(* Logix 5000 AddOnInstructionDefinition export CIP_Axis_Disable; software revision 34.01; part 3 of 4 *)
(* tags used below, declared in another part *)
   StateMachineErrorCode : INT;
   StateMachineErrorDescription : STRING;
   UpdatePeriod : DINT;
   Unwind : DINT;
   AxisControlWord : INT;
   AxisReadyToSwitchOn : BOOL;
   AxisSwitchedOn : BOOL;
   AxisOperationEnabled : BOOL;
   AxisFaulted : BOOL;
   AxisVoltageEnabled : BOOL;
   AxisQuickStop : BOOL;
   AxisSwitchOnDisabled : BOOL;
   AxisWarning : BOOL;
   AxisSTO : BOOL;
   AxisRemote : BOOL;
   AxisTargetReached : BOOL;
   AxisInternalLimitActive : BOOL;
   AxisHomeAttained : BOOL;
   AxisHomingError : BOOL;
   AxisMotionModeHoming : BOOL;
   AxisMotionModeCyclicPosition : BOOL;
   AxisFollowingError : BOOL;
   AxisStreamingActive : BOOL;
   ErrorEnumeratedValues : STRING[13];
   UpdatePeriodMsgSent : BOOL;
   UnwindMsgSent : BOOL;
   IsRotary : SINT;
(* CIP_Axis_State_Machine, continued *)

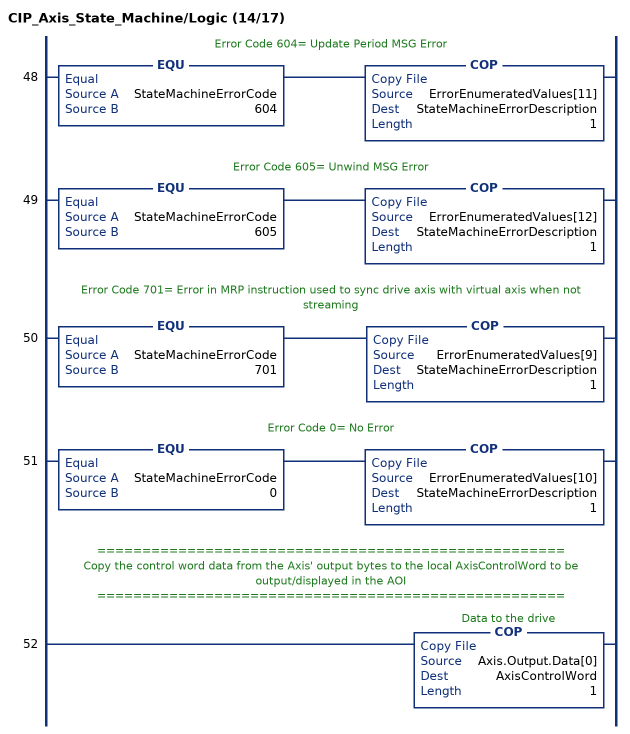
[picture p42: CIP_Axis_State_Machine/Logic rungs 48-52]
   // Error Code 604= Update Period MSG Error
   48: EQU(StateMachineErrorCode,604)COP(ErrorEnumeratedValues[11],StateMachineErrorDescription,1);
   // Error Code 605= Unwind MSG Error
   49: EQU(StateMachineErrorCode,605)COP(ErrorEnumeratedValues[12],StateMachineErrorDescription,1);
   // Error Code 701= Error in MRP instruction used to sync drive axis with virtual axis when not streaming
   50: EQU(StateMachineErrorCode,701)COP(ErrorEnumeratedValues[9],StateMachineErrorDescription,1);
   // Error Code 0= No Error
   51: EQU(StateMachineErrorCode,0)COP(ErrorEnumeratedValues[10],StateMachineErrorDescription,1);
   // ====================================================
   // Copy the control word data from the Axis' output bytes to the local AxisControlWord to be output/displayed in the AOI
   // ====================================================
   52: COP(Axis.Output.Data[0],AxisControlWord,1);
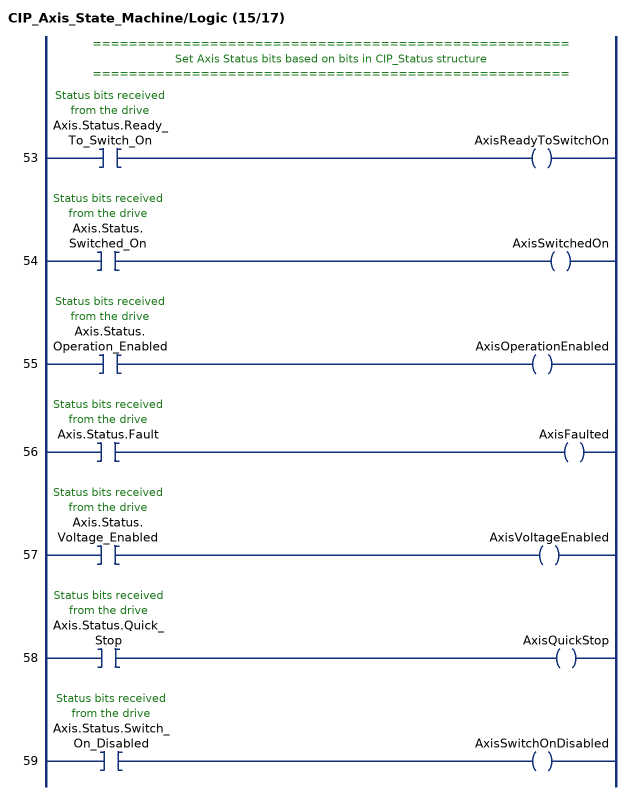
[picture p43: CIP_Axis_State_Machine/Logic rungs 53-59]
   // =====================================================
   // Set Axis Status bits based on bits in CIP_Status structure
   // =====================================================
   53: XIC(Axis.Status.Ready_To_Switch_On)OTE(AxisReadyToSwitchOn);
   54: XIC(Axis.Status.Switched_On)OTE(AxisSwitchedOn);
   55: XIC(Axis.Status.Operation_Enabled)OTE(AxisOperationEnabled);
   56: XIC(Axis.Status.Fault)OTE(AxisFaulted);
   57: XIC(Axis.Status.Voltage_Enabled)OTE(AxisVoltageEnabled);
   58: XIC(Axis.Status.Quick_Stop)OTE(AxisQuickStop);
   59: XIC(Axis.Status.Switch_On_Disabled)OTE(AxisSwitchOnDisabled);
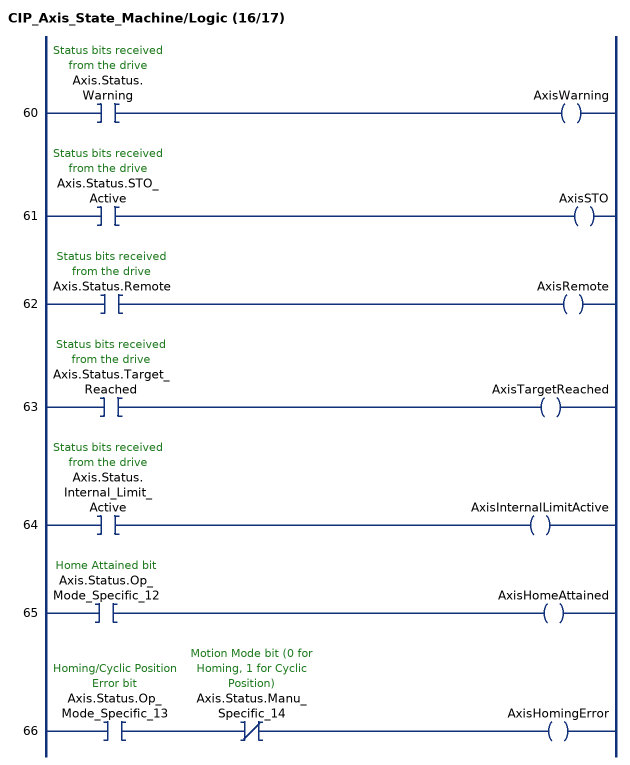
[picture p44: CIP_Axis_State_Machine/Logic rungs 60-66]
   60: XIC(Axis.Status.Warning)OTE(AxisWarning);
   61: XIC(Axis.Status.STO_Active)OTE(AxisSTO);
   62: XIC(Axis.Status.Remote)OTE(AxisRemote);
   63: XIC(Axis.Status.Target_Reached)OTE(AxisTargetReached);
   64: XIC(Axis.Status.Internal_Limit_Active)OTE(AxisInternalLimitActive);
   65: XIC(Axis.Status.Op_Mode_Specific_12)OTE(AxisHomeAttained);
   66: XIC(Axis.Status.Op_Mode_Specific_13)XIO(Axis.Status.Manu_Specific_14)OTE(AxisHomingError);
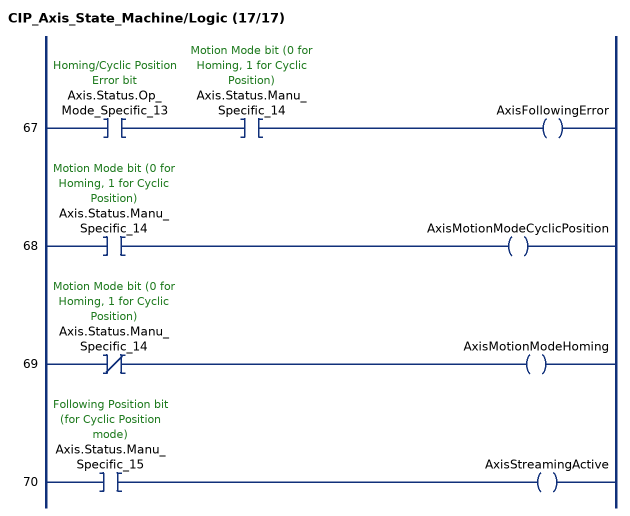
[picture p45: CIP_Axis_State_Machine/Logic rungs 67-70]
   67: XIC(Axis.Status.Op_Mode_Specific_13)XIC(Axis.Status.Manu_Specific_14)OTE(AxisFollowingError);
   68: XIC(Axis.Status.Manu_Specific_14)OTE(AxisMotionModeCyclicPosition);
   69: XIO(Axis.Status.Manu_Specific_14)OTE(AxisMotionModeHoming);
   70: XIC(Axis.Status.Manu_Specific_15)OTE(AxisStreamingActive);
END_ROUTINE

ROUTINE Prescan   (* ladder *)
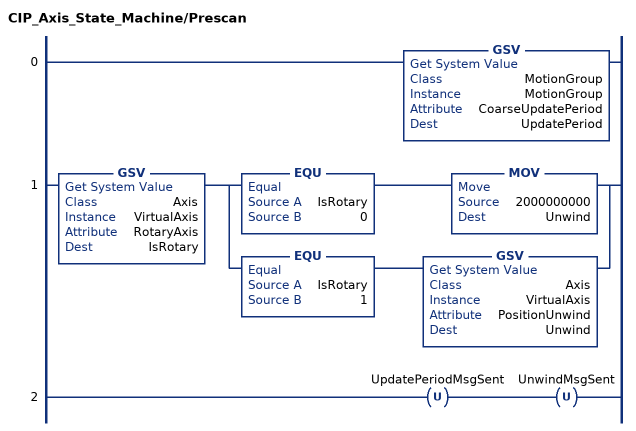
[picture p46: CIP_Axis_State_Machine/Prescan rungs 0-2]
   0: GSV(MotionGroup,MotionGroup,CoarseUpdatePeriod,UpdatePeriod);
   1: GSV(Axis,VirtualAxis,RotaryAxis,IsRotary)[EQU(IsRotary,0) MOV(2000000000,Unwind) ,EQU(IsRotary,1) GSV(Axis,VirtualAxis,PositionUnwind,Unwind) ];
   2: OTU(UpdatePeriodMsgSent)OTU(UnwindMsgSent);
END_ROUTINE
END_ADD_ON_INSTRUCTION

ADD_ON_INSTRUCTION CIP_Drive_Comms_Dual_Axis   (* revision 2.1, ExecutePrescan *)
// CIP Sync Drive Communications For AKD2G Dual Axis Drive
// Revision note:
// Changed local tag CycleStartTime from LINT to DINT[2]. Changed GSV destination and both COP instruction Source entries to use CycleStartTime[0] as a result of the change in data typing.
VAR_IN_OUT
   InputFromDrive : SINT[64]; {required}
   OutputToDrive : SINT[64]; {required}
   Axis1 : CIP_Axis; {required}
   Axis2 : CIP_Axis; {required}
   VirtualAxis1 : AXIS_VIRTUAL; {required}
   VirtualAxis2 : AXIS_VIRTUAL; {required}
   MotionGroup : MOTION_GROUP; {required}
   DynamicMap : CIP_DynamicMap; {required}
END_VAR
VAR
   CycleStartTime : DINT[2]; {access None}
   AxisPosition : DINT; {access None}
END_VAR

ROUTINE Logic   (* ladder *)
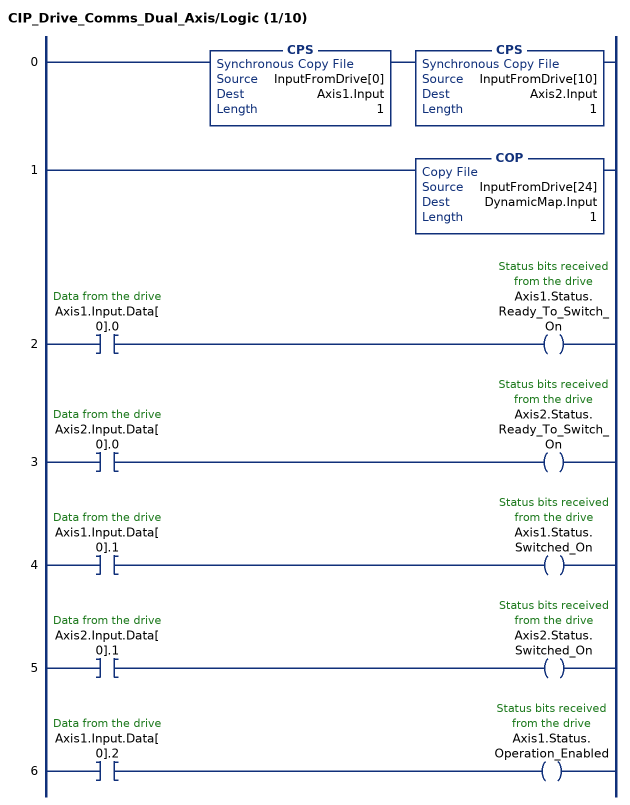
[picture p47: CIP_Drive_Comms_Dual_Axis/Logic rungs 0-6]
   0: CPS(InputFromDrive[0],Axis1.Input,1)CPS(InputFromDrive[10],Axis2.Input,1);
   1: COP(InputFromDrive[24],DynamicMap.Input,1);
   2: XIC(Axis1.Input.Data[0].0)OTE(Axis1.Status.Ready_To_Switch_On);
   3: XIC(Axis2.Input.Data[0].0)OTE(Axis2.Status.Ready_To_Switch_On);
   4: XIC(Axis1.Input.Data[0].1)OTE(Axis1.Status.Switched_On);
   5: XIC(Axis2.Input.Data[0].1)OTE(Axis2.Status.Switched_On);
   6: XIC(Axis1.Input.Data[0].2)OTE(Axis1.Status.Operation_Enabled);
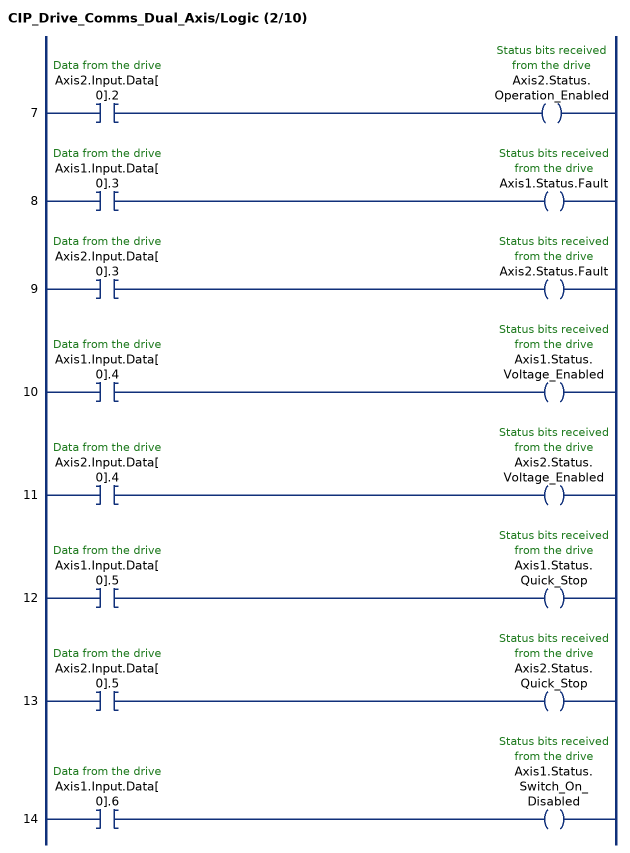
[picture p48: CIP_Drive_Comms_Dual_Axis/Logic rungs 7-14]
   7: XIC(Axis2.Input.Data[0].2)OTE(Axis2.Status.Operation_Enabled);
   8: XIC(Axis1.Input.Data[0].3)OTE(Axis1.Status.Fault);
   9: XIC(Axis2.Input.Data[0].3)OTE(Axis2.Status.Fault);
   10: XIC(Axis1.Input.Data[0].4)OTE(Axis1.Status.Voltage_Enabled);
   11: XIC(Axis2.Input.Data[0].4)OTE(Axis2.Status.Voltage_Enabled);
   12: XIC(Axis1.Input.Data[0].5)OTE(Axis1.Status.Quick_Stop);
   13: XIC(Axis2.Input.Data[0].5)OTE(Axis2.Status.Quick_Stop);
   14: XIC(Axis1.Input.Data[0].6)OTE(Axis1.Status.Switch_On_Disabled);
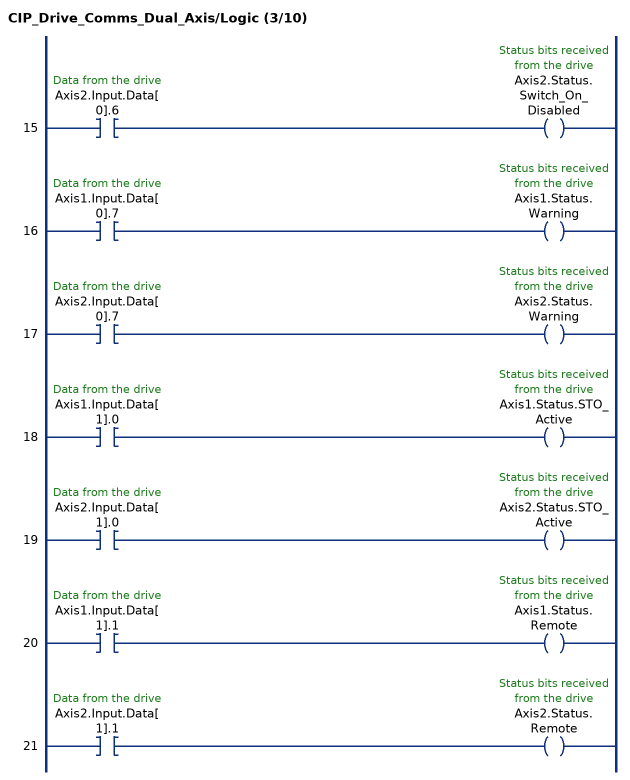
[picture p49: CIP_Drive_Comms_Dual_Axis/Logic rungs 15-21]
   15: XIC(Axis2.Input.Data[0].6)OTE(Axis2.Status.Switch_On_Disabled);
   16: XIC(Axis1.Input.Data[0].7)OTE(Axis1.Status.Warning);
   17: XIC(Axis2.Input.Data[0].7)OTE(Axis2.Status.Warning);
   18: XIC(Axis1.Input.Data[1].0)OTE(Axis1.Status.STO_Active);
   19: XIC(Axis2.Input.Data[1].0)OTE(Axis2.Status.STO_Active);
   20: XIC(Axis1.Input.Data[1].1)OTE(Axis1.Status.Remote);
   21: XIC(Axis2.Input.Data[1].1)OTE(Axis2.Status.Remote);
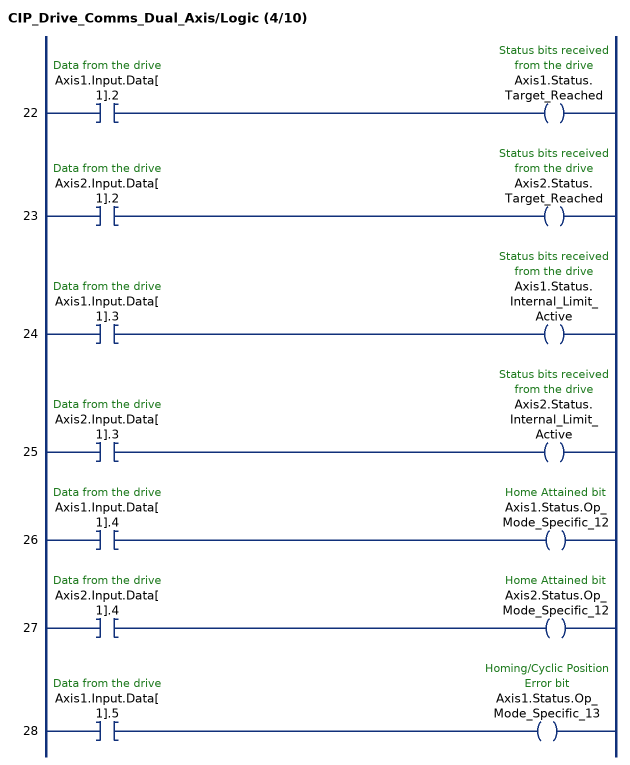
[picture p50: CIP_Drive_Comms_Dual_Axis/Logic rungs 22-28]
   22: XIC(Axis1.Input.Data[1].2)OTE(Axis1.Status.Target_Reached);
   23: XIC(Axis2.Input.Data[1].2)OTE(Axis2.Status.Target_Reached);
   24: XIC(Axis1.Input.Data[1].3)OTE(Axis1.Status.Internal_Limit_Active);
   25: XIC(Axis2.Input.Data[1].3)OTE(Axis2.Status.Internal_Limit_Active);
   26: XIC(Axis1.Input.Data[1].4)OTE(Axis1.Status.Op_Mode_Specific_12);
   27: XIC(Axis2.Input.Data[1].4)OTE(Axis2.Status.Op_Mode_Specific_12);
   28: XIC(Axis1.Input.Data[1].5)OTE(Axis1.Status.Op_Mode_Specific_13);
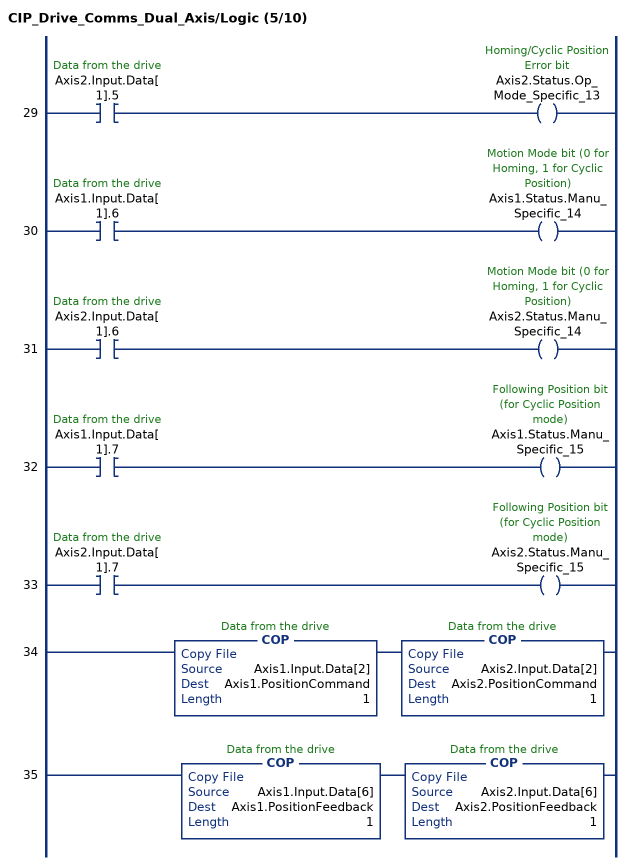
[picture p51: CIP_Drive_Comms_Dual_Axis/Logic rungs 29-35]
   29: XIC(Axis2.Input.Data[1].5)OTE(Axis2.Status.Op_Mode_Specific_13);
   30: XIC(Axis1.Input.Data[1].6)OTE(Axis1.Status.Manu_Specific_14);
   31: XIC(Axis2.Input.Data[1].6)OTE(Axis2.Status.Manu_Specific_14);
   32: XIC(Axis1.Input.Data[1].7)OTE(Axis1.Status.Manu_Specific_15);
   33: XIC(Axis2.Input.Data[1].7)OTE(Axis2.Status.Manu_Specific_15);
   34: COP(Axis1.Input.Data[2],Axis1.PositionCommand,1)COP(Axis2.Input.Data[2],Axis2.PositionCommand,1);
   35: COP(Axis1.Input.Data[6],Axis1.PositionFeedback,1)COP(Axis2.Input.Data[6],Axis2.PositionFeedback,1);
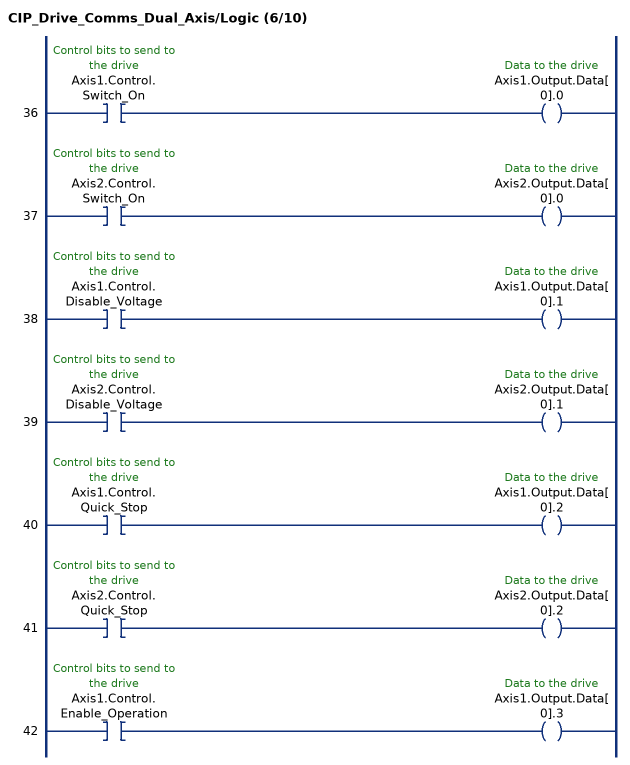
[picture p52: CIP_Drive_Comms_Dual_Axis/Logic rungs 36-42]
   36: XIC(Axis1.Control.Switch_On)OTE(Axis1.Output.Data[0].0);
   37: XIC(Axis2.Control.Switch_On)OTE(Axis2.Output.Data[0].0);
   38: XIC(Axis1.Control.Disable_Voltage)OTE(Axis1.Output.Data[0].1);
   39: XIC(Axis2.Control.Disable_Voltage)OTE(Axis2.Output.Data[0].1);
   40: XIC(Axis1.Control.Quick_Stop)OTE(Axis1.Output.Data[0].2);
   41: XIC(Axis2.Control.Quick_Stop)OTE(Axis2.Output.Data[0].2);
   42: XIC(Axis1.Control.Enable_Operation)OTE(Axis1.Output.Data[0].3);
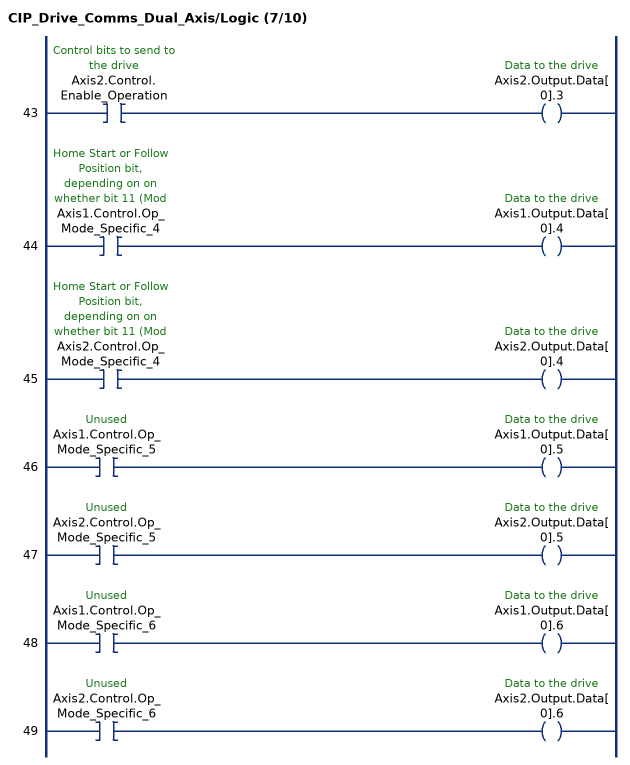
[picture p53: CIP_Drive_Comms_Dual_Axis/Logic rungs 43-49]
   43: XIC(Axis2.Control.Enable_Operation)OTE(Axis2.Output.Data[0].3);
   44: XIC(Axis1.Control.Op_Mode_Specific_4)OTE(Axis1.Output.Data[0].4);
   45: XIC(Axis2.Control.Op_Mode_Specific_4)OTE(Axis2.Output.Data[0].4);
   46: XIC(Axis1.Control.Op_Mode_Specific_5)OTE(Axis1.Output.Data[0].5);
   47: XIC(Axis2.Control.Op_Mode_Specific_5)OTE(Axis2.Output.Data[0].5);
   48: XIC(Axis1.Control.Op_Mode_Specific_6)OTE(Axis1.Output.Data[0].6);
   49: XIC(Axis2.Control.Op_Mode_Specific_6)OTE(Axis2.Output.Data[0].6);
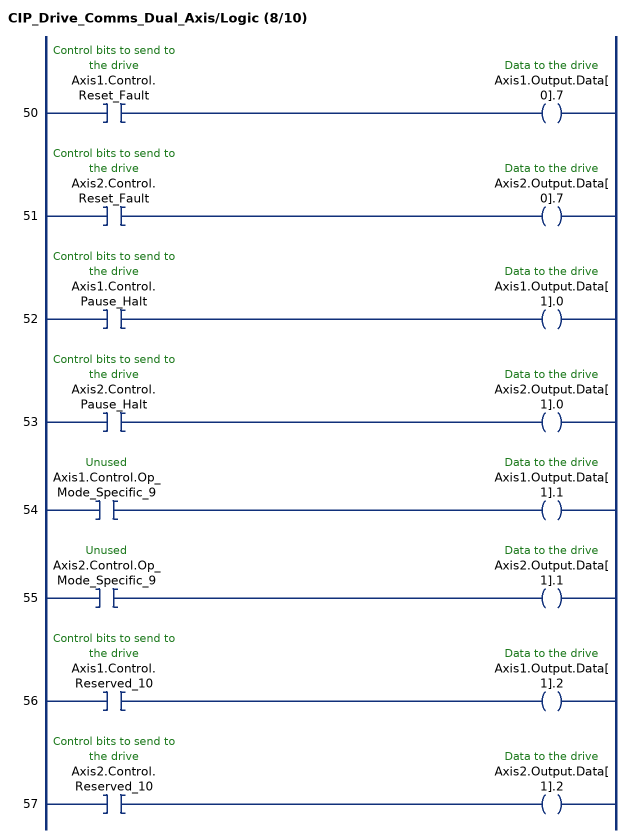
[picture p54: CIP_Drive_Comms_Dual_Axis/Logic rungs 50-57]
   50: XIC(Axis1.Control.Reset_Fault)OTE(Axis1.Output.Data[0].7);
   51: XIC(Axis2.Control.Reset_Fault)OTE(Axis2.Output.Data[0].7);
   52: XIC(Axis1.Control.Pause_Halt)OTE(Axis1.Output.Data[1].0);
   53: XIC(Axis2.Control.Pause_Halt)OTE(Axis2.Output.Data[1].0);
   54: XIC(Axis1.Control.Op_Mode_Specific_9)OTE(Axis1.Output.Data[1].1);
   55: XIC(Axis2.Control.Op_Mode_Specific_9)OTE(Axis2.Output.Data[1].1);
   56: XIC(Axis1.Control.Reserved_10)OTE(Axis1.Output.Data[1].2);
   57: XIC(Axis2.Control.Reserved_10)OTE(Axis2.Output.Data[1].2);
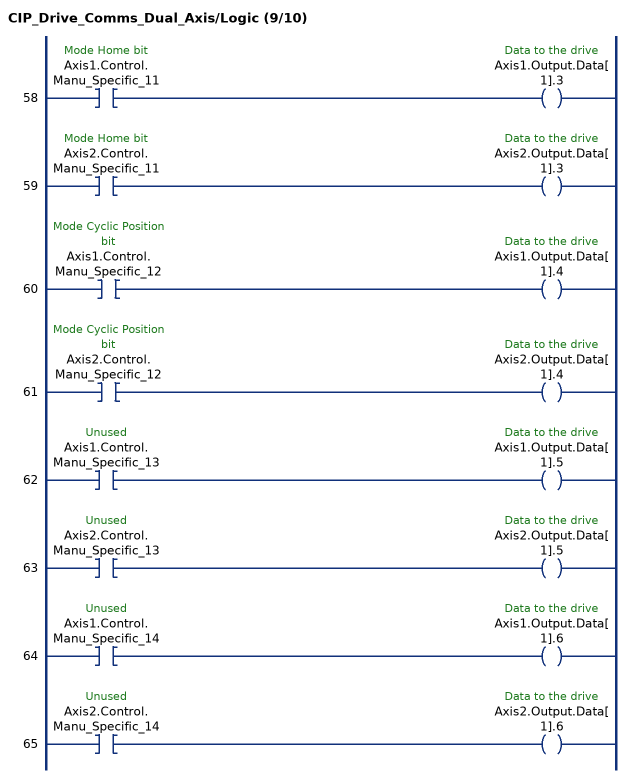
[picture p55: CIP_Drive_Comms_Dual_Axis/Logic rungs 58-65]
   58: XIC(Axis1.Control.Manu_Specific_11)OTE(Axis1.Output.Data[1].3);
   59: XIC(Axis2.Control.Manu_Specific_11)OTE(Axis2.Output.Data[1].3);
   60: XIC(Axis1.Control.Manu_Specific_12)OTE(Axis1.Output.Data[1].4);
   61: XIC(Axis2.Control.Manu_Specific_12)OTE(Axis2.Output.Data[1].4);
   62: XIC(Axis1.Control.Manu_Specific_13)OTE(Axis1.Output.Data[1].5);
   63: XIC(Axis2.Control.Manu_Specific_13)OTE(Axis2.Output.Data[1].5);
   64: XIC(Axis1.Control.Manu_Specific_14)OTE(Axis1.Output.Data[1].6);
   65: XIC(Axis2.Control.Manu_Specific_14)OTE(Axis2.Output.Data[1].6);
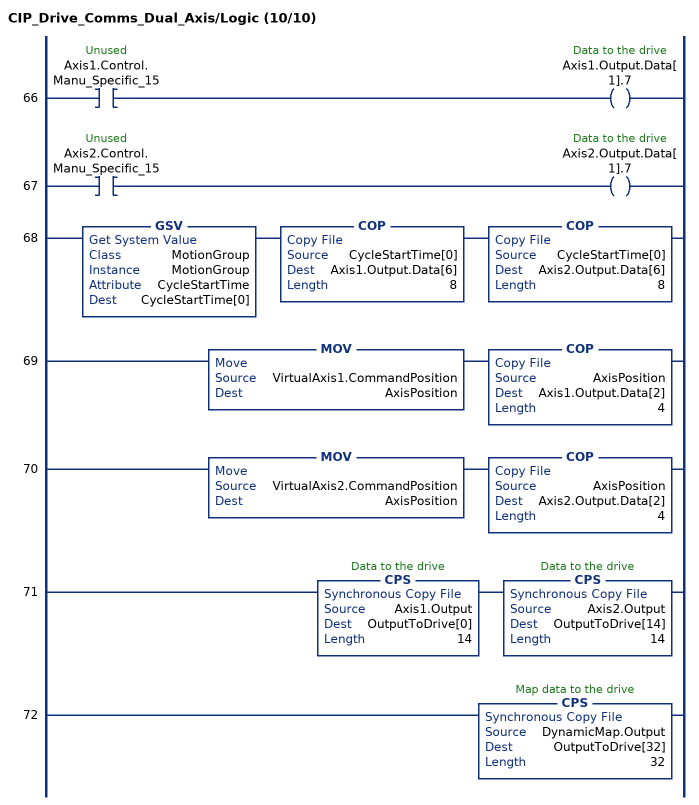
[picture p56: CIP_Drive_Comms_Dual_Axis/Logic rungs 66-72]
   66: XIC(Axis1.Control.Manu_Specific_15)OTE(Axis1.Output.Data[1].7);
   67: XIC(Axis2.Control.Manu_Specific_15)OTE(Axis2.Output.Data[1].7);
   68: GSV(MotionGroup,MotionGroup,CycleStartTime,CycleStartTime[0])COP(CycleStartTime[0],Axis1.Output.Data[6],8)COP(CycleStartTime[0],Axis2.Output.Data[6],8);
   69: MOV(VirtualAxis1.CommandPosition,AxisPosition)COP(AxisPosition,Axis1.Output.Data[2],4);
   70: MOV(VirtualAxis2.CommandPosition,AxisPosition)COP(AxisPosition,Axis2.Output.Data[2],4);
   71: CPS(Axis1.Output,OutputToDrive[0],14)CPS(Axis2.Output,OutputToDrive[14],14);
   72: CPS(DynamicMap.Output,OutputToDrive[32],32);
END_ROUTINE

ROUTINE Prescan   (* ladder *)
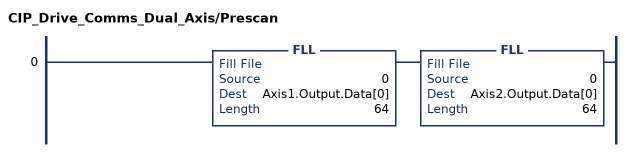
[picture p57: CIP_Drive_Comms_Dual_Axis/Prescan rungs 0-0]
   0: FLL(0,Axis1.Output.Data[0],64)FLL(0,Axis2.Output.Data[0],64);
END_ROUTINE
END_ADD_ON_INSTRUCTION

ADD_ON_INSTRUCTION CIP_Drive_Comms_Single_Axis   (* revision 2.1, ExecutePrescan *)
// CIP Sync Drive Communications For AKD2G Single Axis or Essentials Drive
// Revision note:
// Changed Local Tag CycleStartTime from LINT to DINT[2]
// Modified GSV Destination and COP Source to CycleStartTime[0] in rung 36 to accommodate the change in data typing.
VAR_IN_OUT
   InputFromDrive : SINT[64]; {required}
   OutputToDrive : SINT[64]; {required}
   Axis : CIP_Axis; {required}
   VirtualAxis : AXIS_VIRTUAL; {required}
   MotionGroup : MOTION_GROUP; {required}
   DynamicMap : CIP_DynamicMap; {required}
END_VAR
VAR
   CycleStartTime : DINT[2]; {access None}
   AxisPosition : DINT; {access None}
END_VAR

ROUTINE Logic   (* ladder *)
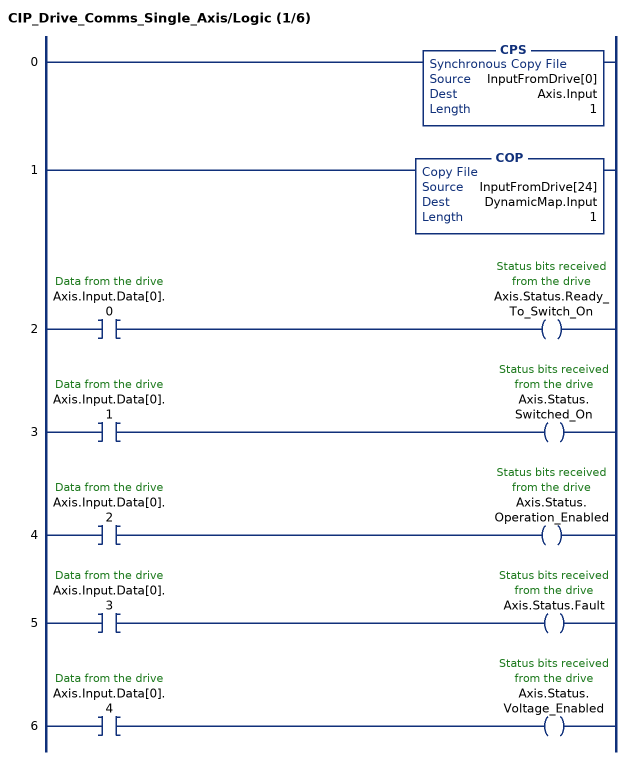
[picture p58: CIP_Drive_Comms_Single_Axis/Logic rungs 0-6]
   0: CPS(InputFromDrive[0],Axis.Input,1);
   1: COP(InputFromDrive[24],DynamicMap.Input,1);
   2: XIC(Axis.Input.Data[0].0)OTE(Axis.Status.Ready_To_Switch_On);
   3: XIC(Axis.Input.Data[0].1)OTE(Axis.Status.Switched_On);
   4: XIC(Axis.Input.Data[0].2)OTE(Axis.Status.Operation_Enabled);
   5: XIC(Axis.Input.Data[0].3)OTE(Axis.Status.Fault);
   6: XIC(Axis.Input.Data[0].4)OTE(Axis.Status.Voltage_Enabled);
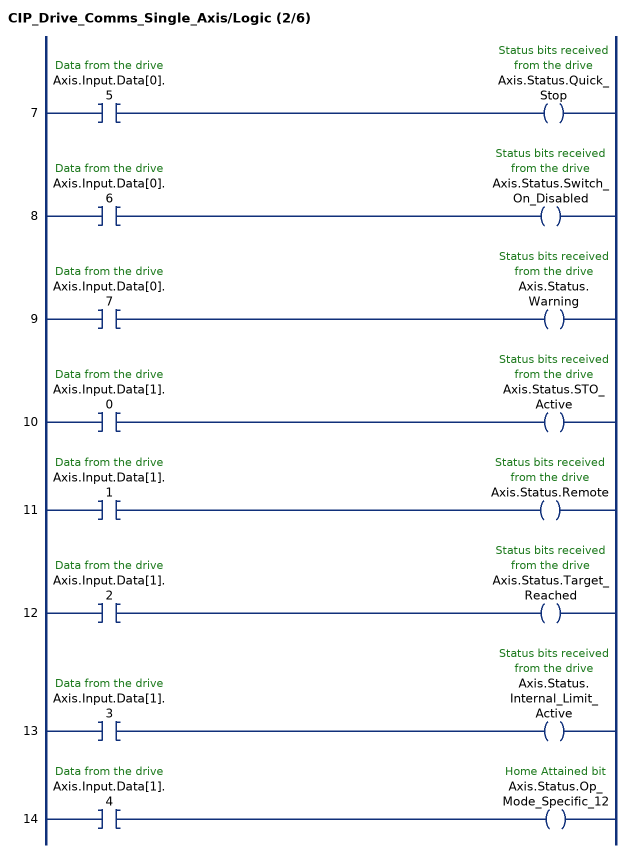
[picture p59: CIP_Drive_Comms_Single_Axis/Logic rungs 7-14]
   7: XIC(Axis.Input.Data[0].5)OTE(Axis.Status.Quick_Stop);
   8: XIC(Axis.Input.Data[0].6)OTE(Axis.Status.Switch_On_Disabled);
   9: XIC(Axis.Input.Data[0].7)OTE(Axis.Status.Warning);
   10: XIC(Axis.Input.Data[1].0)OTE(Axis.Status.STO_Active);
   11: XIC(Axis.Input.Data[1].1)OTE(Axis.Status.Remote);
   12: XIC(Axis.Input.Data[1].2)OTE(Axis.Status.Target_Reached);
   13: XIC(Axis.Input.Data[1].3)OTE(Axis.Status.Internal_Limit_Active);
   14: XIC(Axis.Input.Data[1].4)OTE(Axis.Status.Op_Mode_Specific_12);
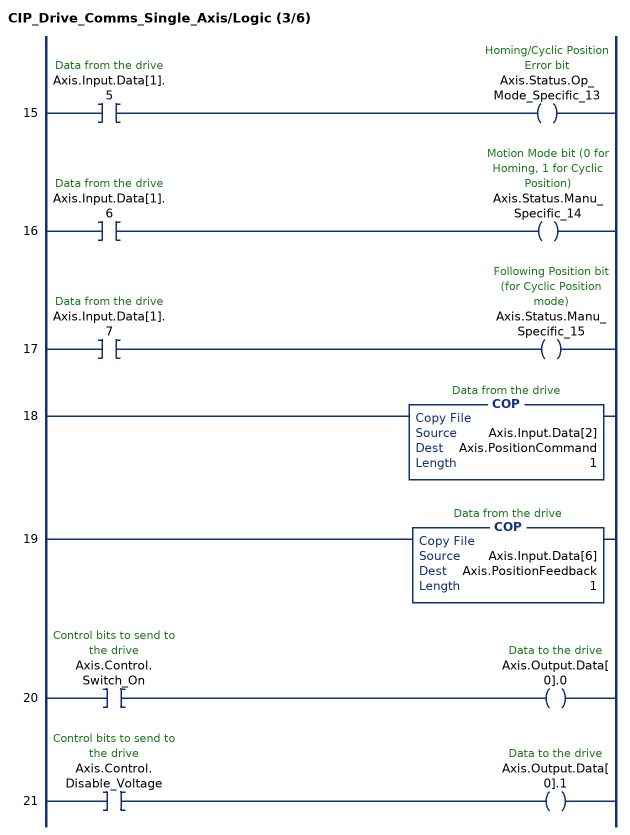
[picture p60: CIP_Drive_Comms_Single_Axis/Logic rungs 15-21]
   15: XIC(Axis.Input.Data[1].5)OTE(Axis.Status.Op_Mode_Specific_13);
   16: XIC(Axis.Input.Data[1].6)OTE(Axis.Status.Manu_Specific_14);
   17: XIC(Axis.Input.Data[1].7)OTE(Axis.Status.Manu_Specific_15);
   18: COP(Axis.Input.Data[2],Axis.PositionCommand,1);
   19: COP(Axis.Input.Data[6],Axis.PositionFeedback,1);
   20: XIC(Axis.Control.Switch_On)OTE(Axis.Output.Data[0].0);
   21: XIC(Axis.Control.Disable_Voltage)OTE(Axis.Output.Data[0].1);
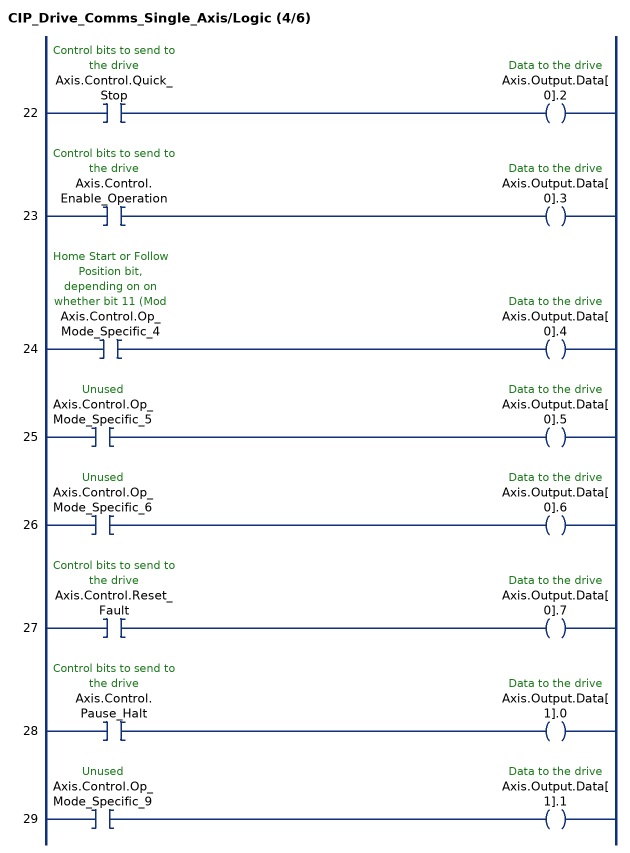
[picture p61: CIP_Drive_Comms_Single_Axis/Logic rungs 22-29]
   22: XIC(Axis.Control.Quick_Stop)OTE(Axis.Output.Data[0].2);
   23: XIC(Axis.Control.Enable_Operation)OTE(Axis.Output.Data[0].3);
   24: XIC(Axis.Control.Op_Mode_Specific_4)OTE(Axis.Output.Data[0].4);
   25: XIC(Axis.Control.Op_Mode_Specific_5)OTE(Axis.Output.Data[0].5);
   26: XIC(Axis.Control.Op_Mode_Specific_6)OTE(Axis.Output.Data[0].6);
   27: XIC(Axis.Control.Reset_Fault)OTE(Axis.Output.Data[0].7);
   28: XIC(Axis.Control.Pause_Halt)OTE(Axis.Output.Data[1].0);
   29: XIC(Axis.Control.Op_Mode_Specific_9)OTE(Axis.Output.Data[1].1);
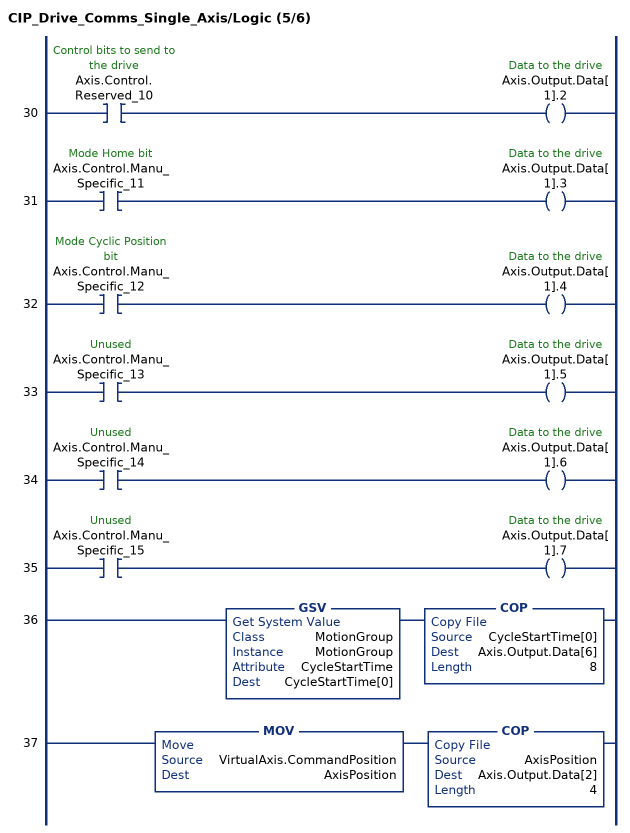
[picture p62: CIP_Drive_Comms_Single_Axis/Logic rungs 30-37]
   30: XIC(Axis.Control.Reserved_10)OTE(Axis.Output.Data[1].2);
   31: XIC(Axis.Control.Manu_Specific_11)OTE(Axis.Output.Data[1].3);
   32: XIC(Axis.Control.Manu_Specific_12)OTE(Axis.Output.Data[1].4);
   33: XIC(Axis.Control.Manu_Specific_13)OTE(Axis.Output.Data[1].5);
   34: XIC(Axis.Control.Manu_Specific_14)OTE(Axis.Output.Data[1].6);
   35: XIC(Axis.Control.Manu_Specific_15)OTE(Axis.Output.Data[1].7);
   36: GSV(MotionGroup,MotionGroup,CycleStartTime,CycleStartTime[0])COP(CycleStartTime[0],Axis.Output.Data[6],8);
   37: MOV(VirtualAxis.CommandPosition,AxisPosition)COP(AxisPosition,Axis.Output.Data[2],4);
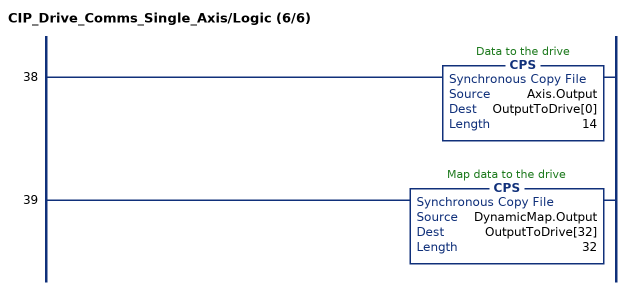
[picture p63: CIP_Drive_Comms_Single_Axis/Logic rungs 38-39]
   38: CPS(Axis.Output,OutputToDrive[0],14);
   39: CPS(DynamicMap.Output,OutputToDrive[32],32);
END_ROUTINE
